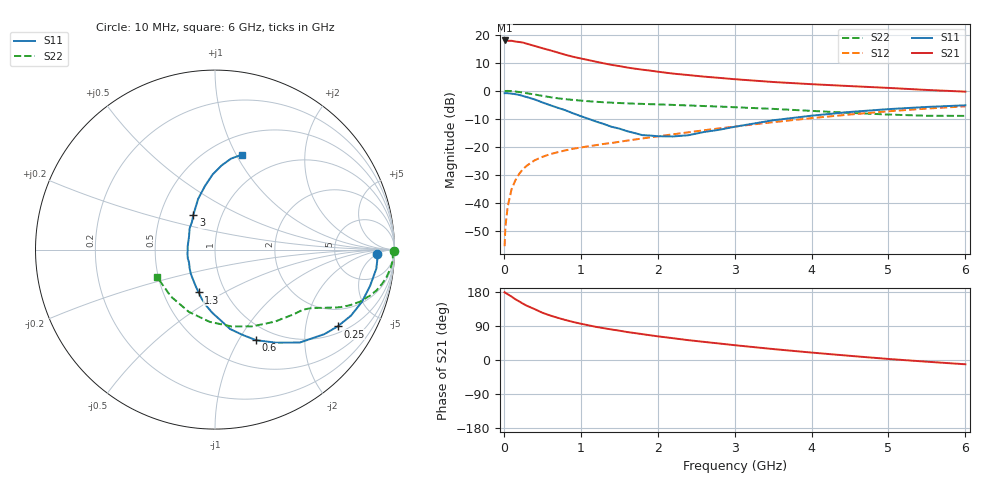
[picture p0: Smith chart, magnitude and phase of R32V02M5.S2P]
! SIEMENS Small Signal Semiconductors
! BFR181
! Si NPN RF Bipolar Junction Transistor in SOT23
! VCE = 2 V  IC = 2.5 mA
! Common Emitter S-Parameters:  May  1996
# GHz  S  MA  R  50
!  f  S11  S21  S12  S22
! GHz  MAG  ANG  MAG  ANG  MAG  ANG  MAG  ANG
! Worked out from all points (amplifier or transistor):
!   36 points, 10 MHz to 6 GHz, reference 50 ohm
!   highest |S21| = 17.9 dB at 10 MHz (marker M1)
!   |S21| within 3 dB of that: start of sweep to 532.8 MHz
!   unconditionally stable (mu >= 1): 1.403 GHz to 3.288 GHz
!   at 250 MHz: K = 0.27, MSG = 22.5 dB, |S12| = -27.9 dB
!   at 1.4 GHz: K = 1.00, MSG = 13.9 dB, |S12| = -18.6 dB
!   at 6 GHz: K = 0.86, MSG = 2.6 dB, |S12| = -5.6 dB
!   S11 on the Smith chart (normalised r, x): 10 MHz: 19, -5; 250 MHz: 1.23, -3.02; 600 MHz: 0.82, -1.19; 1.3 GHz: 0.75, -0.38; 3 GHz: 0.73, +0.30; 6 GHz: 0.70, +1.06
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0.01  0.9056 -1.5  7.875 178.8  0.0017 87.0  0.9962 -0.6
0.02  0.907 -2.8  7.785 177.2  0.0037 84.0  0.9892 -1.3
0.05  0.9049 -6.8  7.768 173.6  0.0086 84.9  0.9932 -3.1
0.1  0.8875 -13.1  7.776 167.4  0.0175 82.5  0.9839 -6.1
0.15  0.8691 -19.5  7.534 160.3  0.0253 78.3  0.9675 -9.2
0.2  0.8423 -25.9  7.389 154.6  0.0331 74.6  0.9492 -11.7
0.25  0.806 -32.1  7.217 148.4  0.0404 72.0  0.9277 -14.2
0.3  0.7702 -37.7  6.88 143.1  0.0464 69.6  0.9026 -16.4
0.4  0.701 -47.6  6.291 134.3  0.0576 64.9  0.8578 -19.8
0.5  0.6206 -56.7  5.733 124.8  0.0662 61.4  0.8115 -22.5
0.6  0.5543 -65.6  5.265 117.6  0.074 59.2  0.7697 -24.6
0.8  0.4498 -79.3  4.376 105.6  0.0866 56.4  0.7075 -27.2
0.9  0.3963 -85.3  4.03 100.4  0.0926 55.4  0.6866 -28.2
1.1  0.3161 -98.9  3.519 91.6  0.1025 55.5  0.6506 -30.0
1.3  0.2555 -111.0  3.079 84.0  0.1129 55.6  0.624 -31.6
1.6  0.1909 -134.8  2.597 73.9  0.1291 56.6  0.5965 -34.1
2.2  0.1533 172.1  2.02 57.5  0.1674 57.5  0.5592 -41.0
3  0.2279 122.0  1.607 39.1  0.2301 55.8  0.5086 -53.3
3.5  0.2977 108.4  1.432 28.9  0.2754 52.9  0.4753 -64.1
4.5  0.419 91.8  1.211 11.0  0.3776 44.0  0.4035 -94.3
5.5  0.5147 80.0  1.033 -4.5  0.4813 31.4  0.3586 -133.3
6  0.5504 74.1  0.964 -11.3  0.5277 24.2  0.3565 -154.4
